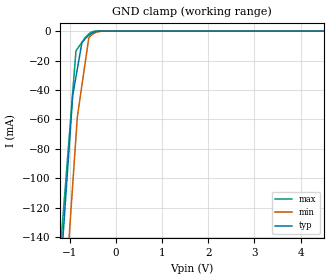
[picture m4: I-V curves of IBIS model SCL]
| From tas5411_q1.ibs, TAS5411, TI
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|   Model
[Model]   SCL
Model_type   Input
Vinl = 0.9
Vinh = 2.31
|   typ   min   max
C_comp   1.263pF   1.204pF   1.431pF
[Voltage Range]   3.3   3   3.6
[Temperature Range]   27   125   -40
[Power Clamp Reference]   3.3   3   3.6
[GND Clamp Reference]   0   0   0
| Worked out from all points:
|   GND clamp passes 1 mA (typ) near -0.50 V on its own axis
[GND Clamp]
|   Voltage   I(typ)   I(min)   I(max)
-3.3V     -1.18A     -1.236A    -1.145A
-1.607V   -351.1mA   -413.7mA   -311.8mA
-933.9mV  -43.68mA   -104mA     -41.35mA
-864.6mV  -31.17mA   -72.11mA   -13.51mA
-834.9mV  -25.81mA   -58.44mA   -12.15mA
-735.9mV  -7.948mA   -36.97mA   -7.635mA
-676.5mV  -5.658mA   -24.09mA   -4.925mA
-587.4mV  -2.91mA    -4.768mA   -2.009mA
-518.1mV  -1.319mA   -2.49mA    -602.1uA
-389.4mV  -95.6uA    -501.1uA   -11.89uA
-191.4mV  -202nA     -7.877uA   0A
6.6V      0A         0A         0A
[POWER Clamp]
|   Voltage   I(typ)   I(min)   I(max)
-3.3V     0A         0A         0A
-3.29V    0A         0A         0A
1.63V     0A         0A         0A
6.6V      0A         0A         0A
